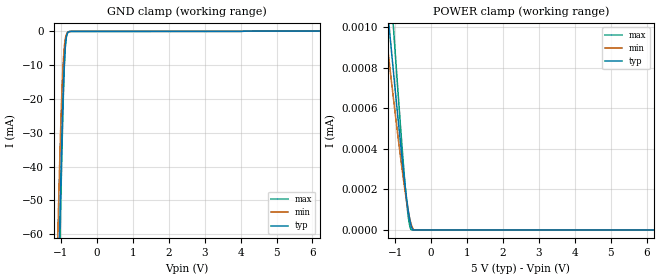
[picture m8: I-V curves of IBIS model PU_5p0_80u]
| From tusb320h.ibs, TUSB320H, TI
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|   Model
[Model]   PU_5p0_80u
Model_type   Input
Vinl = 1.5
Vinh = 3.5
|   typ   min   max
C_comp   0.475pF   0.451pF   0.489pF
[Voltage Range]   5   4.999   5.001
[Temperature Range]   27   105   -40
[Power Clamp Reference]   5   4.999   5.001
[GND Clamp Reference]   0   0   0
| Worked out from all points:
|   GND clamp passes 1 mA (typ) near -0.83 V on its own axis
[GND Clamp]
|   Voltage   I(typ)   I(min)   I(max)
-5V       -2.345A    -2.242A    -2.422A
-1.085V   -81.53mA   -58.82mA   -91.11mA
-1.04V    -59.71mA   -40.13mA   -67.51mA
-1.025V   -52.74mA   -34.4mA    -59.89mA
-995mV    -39.46mA   -23.96mA   -45.17mA
-965mV    -27.35mA   -15.23mA   -31.43mA
-935mV    -16.96mA   -8.654mA   -19.26mA
-905mV    -8.999mA   -4.372mA   -9.613mA
-890mV    -6.114mA   -2.994mA   -6.113mA
-860mV    -2.483mA   -1.345mA   -1.995mA
-800mV    -353.5uA   -286.7uA   -205.6uA
10V       0A         0A         0A
[POWER Clamp]
|   Voltage   I(typ)   I(min)   I(max)
-5V       8.523uA    1.593A     11.61uA
-1.91V    2.427uA    87.48uA    3.265uA
-1.25V    1.158uA    959.6nA    1.521uA
-1.145V   960.8nA    797.1nA    1.249uA
-1.04V    766.4nA    637.3nA    979.9nA
-830mV    392.3nA    332.2nA    461.8nA
-695mV    176.2nA    158.2nA    166.7nA
-650mV    114.5nA    108.4nA    88.13nA
-605mV    62.54nA    65.62nA    31.31nA
-530mV    8.341nA    15.64nA    0A
-485mV    0A         0A         0A
10V       0A         0A         0A
